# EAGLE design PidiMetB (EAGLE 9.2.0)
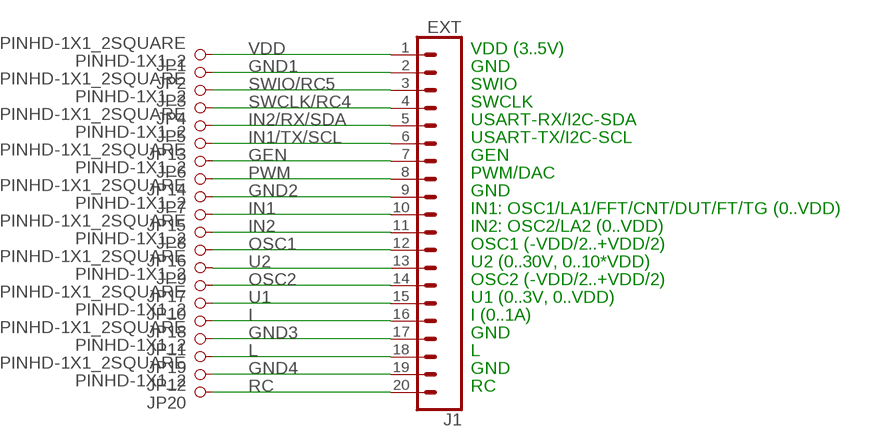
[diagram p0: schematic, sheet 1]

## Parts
J1  EXT  CONN_201X20_LONGPADS  [1X20_LONGPADS]
JP1  PINHD-1X1_2SQUARE  [1X1-BIG2]
JP2  PINHD-1X1_2  [1X1-BIG]
JP3  PINHD-1X1_2SQUARE  [1X1-BIG2]
JP4  PINHD-1X1_2  [1X1-BIG]
JP5  PINHD-1X1_2SQUARE  [1X1-BIG2]
JP6  PINHD-1X1_2SQUARE  [1X1-BIG2]
JP7  PINHD-1X1_2SQUARE  [1X1-BIG2]
JP8  PINHD-1X1_2SQUARE  [1X1-BIG2]
JP9  PINHD-1X1_2SQUARE  [1X1-BIG2]
JP10  PINHD-1X1_2SQUARE  [1X1-BIG2]
JP11  PINHD-1X1_2SQUARE  [1X1-BIG2]
JP12  PINHD-1X1_2SQUARE  [1X1-BIG2]
JP13  PINHD-1X1_2  [1X1-BIG]
JP14  PINHD-1X1_2  [1X1-BIG]
JP15  PINHD-1X1_2  [1X1-BIG]
JP16  PINHD-1X1_2  [1X1-BIG]
JP17  PINHD-1X1_2  [1X1-BIG]
JP18  PINHD-1X1_2  [1X1-BIG]
JP19  PINHD-1X1_2  [1X1-BIG]
JP20  PINHD-1X1_2  [1X1-BIG]

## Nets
GEN: J1.7 JP6.P$1
GND1: J1.2 JP2.P$1
GND2: J1.9 JP7.P$1
GND3: J1.17 JP11.P$1
GND4: J1.19 JP12.P$1
I: J1.16 JP18.P$1
IN1: J1.10 JP15.P$1
IN1/TX/SCL: J1.6 JP13.P$1
IN2: J1.11 JP8.P$1
IN2/RX/SDA: J1.5 JP5.P$1
L: J1.18 JP19.P$1
OSC1: J1.12 JP16.P$1
OSC2: J1.14 JP17.P$1
PWM: J1.8 JP14.P$1
RC: J1.20 JP20.P$1
SWCLK/RC4: J1.4 JP4.P$1
SWIO/RC5: J1.3 JP3.P$1
U1: J1.15 JP10.P$1
U2: J1.13 JP9.P$1
VDD: J1.1 JP1.P$1

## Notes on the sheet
- VDD (3..5V)
- GND
- SWIO
- SWCLK
- USART-RX/I2C-SDA
- USART-TX/I2C-SCL
- GEN
- PWM/DAC
- GND
- IN1: OSC1/LA1/FFT/CNT/DUT/FT/TG (0..VDD)
- IN2: OSC2/LA2 (0..VDD)
- OSC1 (-VDD/2..+VDD/2)
- U2 (0..30V, 0..10*VDD)
- OSC2 (-VDD/2..+VDD/2)
- U1 (0..3V, 0..VDD)
- I (0..1A)
- GND
- L
- GND
- RC

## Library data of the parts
J1 = SparkFun-Connectors:CONN_20: Multi connection point. Often used as Generic Header-pin footprint for 0.1 inch spaced/style header connections On any of the 0.1 inch spaced packages, you can populate with these: Break Away Headers - Straight (PRT-00116) Break Away Male Headers - Right Angle (PRT-00553) Female Headers (PRT-00115)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
JP1-JP20 = adafruit:PINHD-1X1_2

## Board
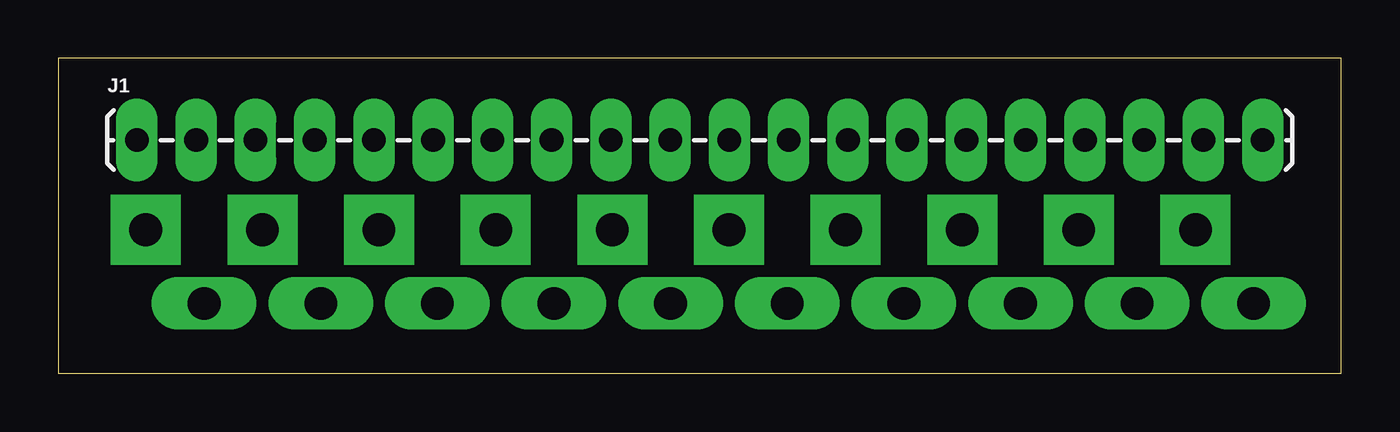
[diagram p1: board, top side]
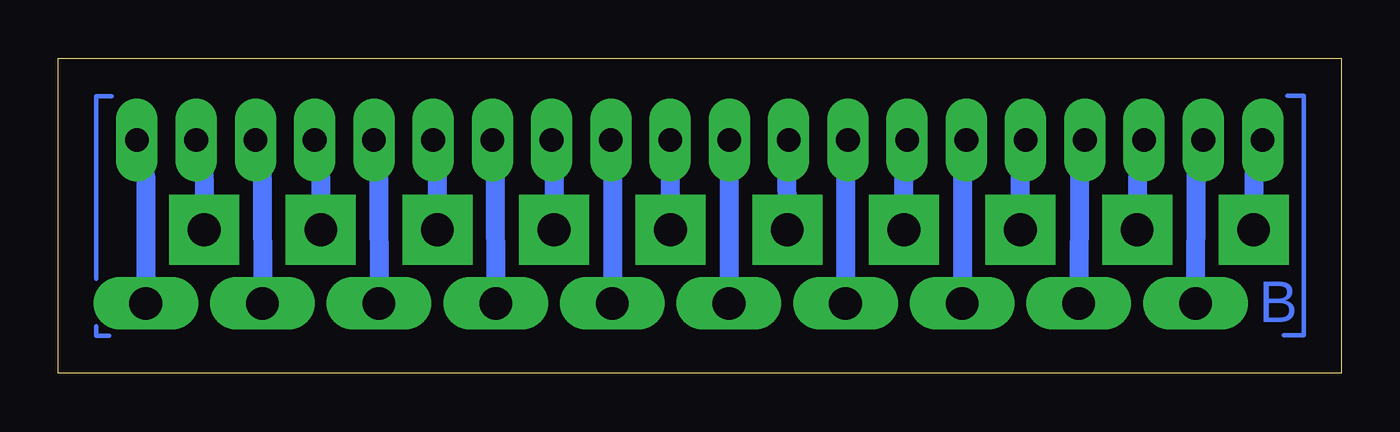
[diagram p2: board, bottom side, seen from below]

Size 55 x 13.5 mm. Coordinates in mm from the lower left corner, seen from the top.
Outline: 0,0 55,0 55,13.5 0,13.5 0,0
Copper layers (1*16): Top 0.035mm / dielectric 1.5mm / Bottom 0.035mm
Design rules "default": minimum track width 6mil, minimum drill 0.35mm, track to track 6mil, track to pad 6mil, pad to pad 6mil, via to via 6mil, smd to smd 6mil, copper to edge 40mil, drill to drill 6mil, minimum pad ring 10mil, minimum via ring 8mil, stop-mask expansion 4mil, vias tented up to drill 0mil, thermal gap 10mil

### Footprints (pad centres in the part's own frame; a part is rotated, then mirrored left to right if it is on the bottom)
1X20_LONGPADS = drill 1.016 pad 1.778 long: 1 -24.13,0; 2 -21.59,0; 3 -19.05,0; 4 -16.51,0; 5 -13.97,0; 6 -11.43,0; 7 -8.89,0; 8 -6.35,0; 9 -3.81,0; 10 -1.27,0; 11 1.27,0; 12 3.81,0; 13 6.35,0; 14 8.89,0; 15 11.43,0; 16 13.97,0; 17 16.51,0; 18 19.05,0; 19 21.59,0; 20 24.13,0
1X1-BIG2 = drill 1.4 pad 3 square: P$1 0,0
1X1-BIG = drill 1.4 pad 2.25 long: P$1 0,0

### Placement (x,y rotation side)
J1  27.5,10 0 top
JP1  3.75,6.15 90 top
JP2  6.25,3 0 top
JP3  8.75,6.15 90 top
JP4  11.25,3 0 top
JP5  13.75,6.15 90 top
JP6  18.75,6.15 0 top
JP7  23.75,6.15 0 top
JP8  28.75,6.15 0 top
JP9  33.75,6.15 0 top
JP10  38.75,6.15 0 top
JP11  43.75,6.15 0 top
JP12  48.75,6.15 0 top
JP13  16.25,3 0 top
JP14  21.25,3 0 top
JP15  26.25,3 0 top
JP16  31.25,3 0 top
JP17  36.25,3 0 top
JP18  41.25,3 0 top
JP19  46.25,3 0 top
JP20  51.25,3 0 top

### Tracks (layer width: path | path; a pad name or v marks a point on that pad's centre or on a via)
GEN
  Bottom 0.813: J1.7 18.77,8.4 JP6.P$1
GND1
  Bottom 0.813: J1.2 6.22,8.45 JP2.P$1
GND2
  Bottom 0.813: J1.9 23.78,8.31 JP7.P$1
GND3
  Bottom 0.813: J1.17 43.75,8.31 JP11.P$1
GND4
  Bottom 0.813: J1.19 48.75,8.36 JP12.P$1
I
  Bottom 0.813: J1.16 41.27,8.36 JP18.P$1
IN1
  Bottom 0.813: J1.10 26.24,8.38 JP15.P$1
IN1/TX/SCL
  Bottom 0.813: J1.6 16.23,8.5 JP13.P$1
IN2
  Bottom 0.813: J1.11 28.77,8.22 JP8.P$1
IN2/RX/SDA
  Bottom 0.813: J1.5 13.77,8.47 JP5.P$1
L
  Bottom 0.813: J1.18 46.26,8.43 JP19.P$1
N$1
  Bottom 0.2: 2.3,11.89 1.6,11.89 1.61,1.63 2.46,1.64
N$2
  Bottom 0.2: 52.7,11.87 53.37,11.88 53.37,4.06
N$3
  Bottom 0.2: 53.37,2.02 53.37,1.62 52.82,1.62
OSC1
  Bottom 0.813: J1.12 31.24,8.31 JP16.P$1
OSC2
  Bottom 0.813: J1.14 36.27,8.45 JP17.P$1
PWM
  Bottom 0.813: J1.8 21.25,8.33 JP14.P$1
RC
  Bottom 0.813: J1.20 51.26,8.47 JP20.P$1
SWCLK/RC4
  Bottom 0.813: J1.4 11.22,8.4 JP4.P$1
SWIO/RC5
  Bottom 0.813: J1.3 8.73,8.36 JP3.P$1
U1
  Bottom 0.813: J1.15 38.76,8.31 JP10.P$1
U2
  Bottom 0.813: J1.13 33.74,8.31 JP9.P$1
VDD
  Bottom 0.813: J1.1 3.74,8.54 JP1.P$1

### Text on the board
Bottom: B
Document: VDD | SWIO | RX/SDA | GEN | GND | IN2 | U2 | U1 | GND | GND | 6 | 10 | 16 | 18 | 20 | 1 | 2 | GND | 3 | 4 | SWCLK | 5 | TX/SCL | 7 | 8 | PWM | 9 | IN1 | 11 | 12 | OSC1 | 13 | 14 | OSC2 | 15 | I | 17 | L | 19 | RC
